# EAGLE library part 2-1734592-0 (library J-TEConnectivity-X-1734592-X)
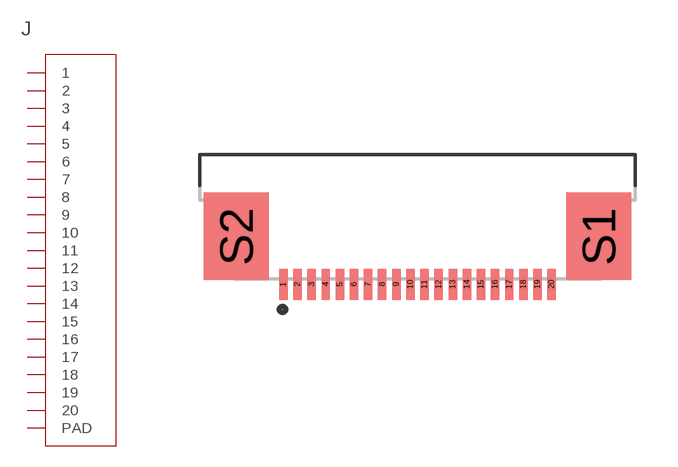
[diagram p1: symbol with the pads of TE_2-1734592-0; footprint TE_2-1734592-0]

Designator prefix J

## 2-1734592-0  [TE_2-1734592-0]
1  1  pas
2  2  pas
3  3  pas
4  4  pas
5  5  pas
6  6  pas
7  7  pas
8  8  pas
9  9  pas
10  10  pas
11  11  pas
12  12  pas
13  13  pas
14  14  pas
15  15  pas
16  16  pas
17  17  pas
18  18  pas
19  19  pas
20  20  pas
S1  PAD
S2  PAD

## Footprint TE_2-1734592-0 (pad centres in mm)
smd 0.3 x 1.1: 1 -4.75,0; 2 -4.25,0; 3 -3.75,0; 4 -3.25,0; 5 -2.75,0; 6 -2.25,0; 7 -1.75,0; 8 -1.25,0; 9 -0.75,0; 10 -0.25,0; 11 0.25,0; 12 0.75,0; 13 1.25,0; 14 1.75,0; 15 2.25,0; 16 2.75,0; 17 3.25,0; 18 3.75,0; 19 4.25,0; 20 4.75,0
smd 2.3 x 3.1: S1 6.42,1.7; S2 -6.42,1.7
